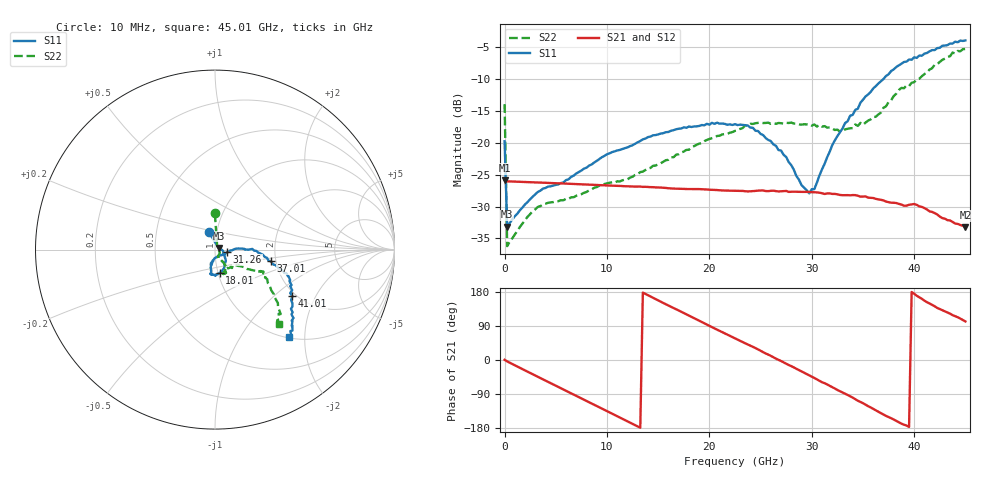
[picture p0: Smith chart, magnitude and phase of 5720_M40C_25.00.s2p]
! Device:  ADRF5720
! Description: 0.5dB LSB GaAs MMIC 6-bit Digital Attenuator
! Frequency:  0.000009 -  40 GHz
! Ports:
!	RF1	= Port 1
!	RF2	= Port 2
! Vdd:  3.3 Volt
! Vss:  -3.3 Volt
! Control:  0/3.3 Volt
! State:  25.00 dB attenuation
! Data:  The device was measured using G-S-G Probes on a matrix board.
!  Data was collected using an calibrated 4 port network analyzer.
!  The reference plane for this measurement is at the launchers.
! Note:  Analog Devices supplies this data as a sample of measured data
!  for this product.  Your particular data for this product may vary.
!  Data was taken at -40 degrees C.
!  Analog Devices reserves the right to change this data at anytime.
# GHZ S DB R 45.0
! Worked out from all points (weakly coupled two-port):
!   181 points, 10 MHz to 45.01 GHz, reference 45 ohm
!   highest |S21| = -25.87 dB at 10 MHz (marker M1); lowest = -33.2 dB at 45.01 GHz (marker M2)
!   lowest |S11| = -33.2 dB at 260 MHz (marker M3), VSWR 1.04, Z = 46.8 + j0.914 ohm
!   |S11| at or under -10 dB: start of sweep to 36.98 GHz
!   |S22| runs from -36.2 to -5.2 dB; largest |S21 - S12| = 0.00024
!   S11 on the Smith chart (normalised r, x): 10 MHz: 0.92, +0.18; 18.01 GHz: 1.02, -0.27; 31.26 GHz: 1.14, -0.03; 37.01 GHz: 1.88, -0.27; 41.01 GHz: 1.91, -1.33; 45.01 GHz: 1.02, -1.67
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0.01  -19.75 109.5  -25.87 0.4  -25.90 0.4  -13.91 90.3
0.26  -33.17 26.4  -26.05 -3.7  -26.07 -3.7  -36.23 32.3
3.26  -27.71 -4.6  -26.23 -44.5  -26.25 -44.5  -30.06 -32.7
7.76  -24.05 -32.4  -26.52 -104.8  -26.54 -104.8  -27.84 -65.7
15.26  -18.53 -67.0  -27.02 153.9  -27.03 153.8  -23.20 -59.6
18.01  -17.43 -78.9  -27.25 117.3  -27.27 117.3  -21.08 -56.9
22.76  -17.20 -99.0  -27.54 53.9  -27.57 53.8  -18.01 -63.3
24.26  -17.63 -100.1  -27.58 34.7  -27.60 34.6  -17.02 -64.8
26.01  -19.71 -103.6  -27.53 10.9  -27.55 10.8  -17.00 -67.7
27.51  -22.21 -101.8  -27.55 -10.0  -27.57 -10.1  -16.84 -70.2
29.01  -26.64 -90.3  -27.70 -30.1  -27.72 -30.2  -17.13 -71.8
29.76  -27.92 -63.3  -27.72 -40.6  -27.74 -40.7  -17.06 -71.8
30.26  -27.27 -42.3  -27.76 -47.5  -27.78 -47.6  -17.10 -70.3
31.26  -23.30 -11.5  -28.03 -61.2  -28.06 -61.4  -17.36 -66.2
33.26  -16.88 2.3  -28.21 -88.7  -28.23 -88.8  -17.88 -54.9
35.01  -13.22 -1.5  -28.44 -113.9  -28.47 -114.0  -17.16 -40.3
37.01  -9.95 -11.8  -29.04 -144.0  -29.07 -144.2  -14.48 -31.1
37.76  -8.70 -16.1  -29.39 -153.7  -29.41 -153.8  -13.31 -30.3
38.76  -7.56 -18.4  -29.69 -168.0  -29.70 -168.2  -11.36 -27.1
41.01  -5.97 -31.0  -30.25 156.6  -30.27 156.6  -9.18 -32.2
43.76  -4.39 -44.5  -32.42 118.4  -32.44 118.0  -5.80 -44.5
45.01  -3.90 -49.7  -33.25 101.8  -33.28 101.6  -5.24 -49.6
